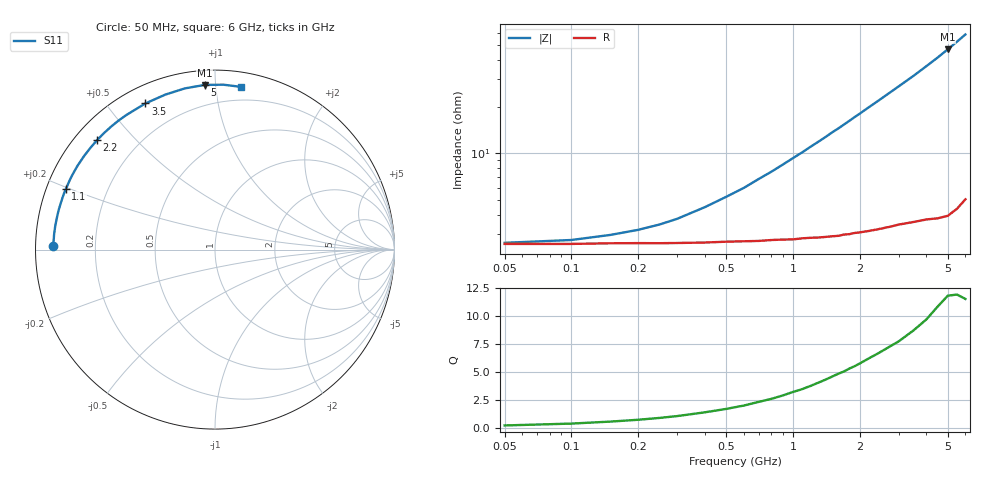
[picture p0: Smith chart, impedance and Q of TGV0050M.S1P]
! SIEMENS Discrete & RF Semiconductors
! BAT64
! Si Schottky Diode in SOT23
! IF = 50 mA
! S-Parameters:  February  1997
# GHz  S  MA  R  50
!  f  S11
! GHz  MAG  ANG
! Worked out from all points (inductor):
!   34 points, 50 MHz to 6 GHz, reference 50 ohm
!   read as one part to ground: L = 1.41 nH near 1 GHz
!   highest Q = 11.9 at 5 GHz (marker M1), where L = 1.49 nH
!   S11 on the Smith chart (normalised r, x): 50 MHz: 0.05, +0.01; 1.1 GHz: 0.06, +0.19; 2.2 GHz: 0.06, +0.39; 3.5 GHz: 0.07, +0.63; 5 GHz: 0.08, +0.94; 6 GHz: 0.10, +1.17
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0.05  0.9012 178.9
0.25  0.9004 174.8
0.4  0.8997 171.7
0.5  0.8988 169.7
0.6  0.8985 167.8
0.7  0.8984 165.7
0.8  0.8976 163.8
1  0.8977 159.8
1.1  0.8968 157.9
1.2  0.8967 155.9
1.3  0.897 154.0
1.4  0.897 152.1
1.5  0.8969 150.1
1.6  0.8971 148.3
1.8  0.8966 144.5
1.9  0.8959 142.6
2  0.8961 140.8
2.2  0.8964 137.1
2.4  0.8966 133.6
2.6  0.897 130.1
2.8  0.8975 126.7
3  0.898 123.4
3.5  0.9019 115.5
4  0.9068 107.8
4.5  0.9137 100.6
5  0.9193 93.6
5.5  0.9199 87.1
6  0.9182 81.0
